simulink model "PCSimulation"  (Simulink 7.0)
settings: Solver=FixedStepDiscrete  SolverMode=SingleTasking  StartTime=0.0  StopTime=inf  FixedStep=samplePeriod  RelTol=1e-3  AbsTol=1e-6
PreLoadFcn:
  | initialize
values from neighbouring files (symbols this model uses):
  acal = acal(:)    [initialize.m]
  actParams = [	bulkModulus   * pressCanon    [initialize.m]
  atype = ones(nact, 1)    [dampmatrix.m]    (also in displA2T.m = []; displEnvelope.m = varargin{1}{6}; displJacobian.m; displT2A.m = [])
  dcal = dcal(:)    [initialize.m]
  fcal = fcal(:)    [initialize.m]
  forceCanon = 0.00444822    [initialize.m]
  inertia = inertia + inertiaP2Q([0 0 0], massA(i), cgA(:,i)-cg,  									inertiaCanon, massCanon)    [initialize.m]
  inertiaMask = zeros(3, 1)    [initialize.m]
  lengthCanon = 25.4    [initialize.m]
  mass = ones(3, 1) * (sum(massA) + massT + massS)    [initialize.m]
  massMask = zeros(3, 1)    [initialize.m]
  nAct = self.nAct    [animation.m]    (also in initialize.m = size(rh, 2))
  nAdcU = 6    [initialize.m]
  nTbl = length(dof)    [initialize.m]
  nUDPInp = 1+nTbl+2*nAct+nAcc+nAdcU    [initialize.m]
  nUDPOut = 1+5*nTbl+nAct+nAdcU    [initialize.m]
  returnPress = 50    [initialize.m]
  rtg = cg    [initialize.m]
  samplePeriod = controlPeriod/upsampleFactor    (= 0.00048828125)    [initialize.m]    (also in viewer.m = eval(getHeaderValue(header, 'DELTA_T')))
  staticForce = forceT2A(ftbl, dtbl0, dof, rh, rb, rl, canon, atype)    [initialize.m]
  upsampleFactor = 1    [initialize.m]
  x = []    [loadbin.m]    (also in quake.m = 365; viewer.m = 40; player.m = xPanel + panelWide + margin; resondemo.m = xOrigin + marginWide + panelWide + plotMarginWide)
undefined symbols (not defined in the file or in its folder): animation, DiscIntNeverNeededParam, friction, yieldDispl
libraries: LibDynamics x12, LibTransforms x12

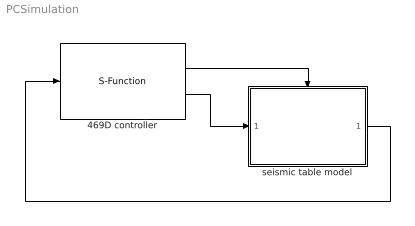
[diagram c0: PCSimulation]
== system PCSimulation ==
  469D controller : S-Function  FunctionName=UDPSimulink  Parameters=5002,nUDPInp,nUDPOut,upsampleFactor
  seismic table model : Subsystem  TreatAsAtomicUnit=on
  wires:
  469D controller/2 -> seismic table model/1(inp)
  469D controller/1 -> seismic table model/Trigger
  seismic table model/1(out) -> 469D controller/1

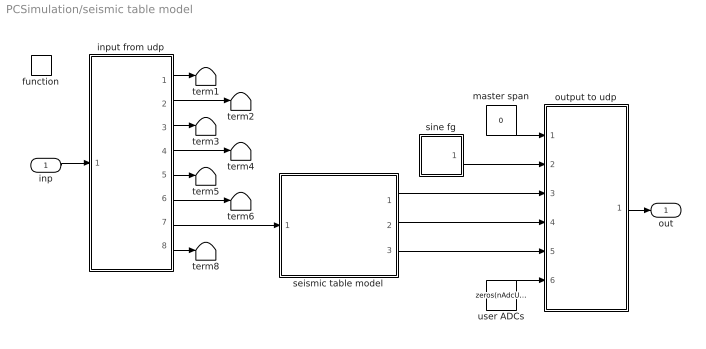
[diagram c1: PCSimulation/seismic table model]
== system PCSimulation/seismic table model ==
  inp : Inport  OutDataType=sfix(16)  OutScaling=2^0
  function : TriggerPort  TriggerType=function-call
  input from udp : Subsystem
  master span : Constant  Value=0  OutDataType=sfix(16)  OutScaling=2^0
  output to udp : Subsystem
  seismic table model : Subsystem
  sine fg : Subsystem  mask(Sine Function Generator){id=x, ampl=0.3, freq=4, phase=0, spanInterval=1, samplePeriod=-1}
      mask prompts: id "DOF"; ampl "Amplitude"; freq "Frequency (Hz)"; phase "Phase (deg)"; spanInterval "Span interval (sec)"; samplePeriod "Sample period (sec)"
  term{1..6,8} (7 alike) : Terminator
  user ADCs : Constant  Value=zeros(nAdcU, 1)  OutDataType=sfix(16)  OutScaling=2^0
  out : Outport  OutDataType=sfix(16)  OutScaling=2^0
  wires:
  input from udp/1(master span) -> term1/1
  input from udp/2(ref) -> term2/1
  input from udp/3(displ fbk) -> term3/1
  input from udp/4(veloc fbk) -> term4/1
  input from udp/5(accel fbk) -> term5/1
  input from udp/6(force fbk) -> term6/1
  input from udp/8(user adcs) -> term8/1
  input from udp/7(valve cmd) -> seismic table model/1(valve cmd)
  inp/1 -> input from udp/1(inp)
  output to udp/1(out) -> out/1
  user ADCs/1 -> output to udp/6(user adcs)
  master span/1 -> output to udp/1(master span)
  seismic table model/1(displ) -> output to udp/3(displ fbk)
  seismic table model/2(accel) -> output to udp/4(accel fbks)
  seismic table model/3(force) -> output to udp/5(force fbk)
  sine fg/1(out) -> output to udp/2(ref)

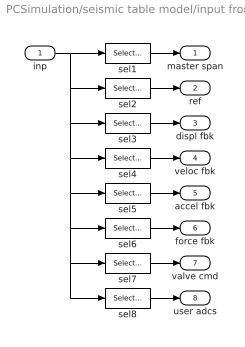
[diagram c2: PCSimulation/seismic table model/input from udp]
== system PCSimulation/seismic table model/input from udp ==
  inp : Inport  OutDataType=sfix(16)  OutScaling=2^0
  sel1 : Selector  InputPortWidth=nUDPOut  IndexOptions=Index vector (dialog)  Indices=[0]+1  OutputSizes=1
  sel2 : Selector  InputPortWidth=nUDPOut  IndexOptions=Index vector (dialog)  Indices=[1:nTbl]+1  OutputSizes=1
  sel3 : Selector  InputPortWidth=nUDPOut  IndexOptions=Index vector (dialog)  Indices=(1:nTbl)+nTbl+1  OutputSizes=1
  sel4 : Selector  InputPortWidth=nUDPOut  IndexOptions=Index vector (dialog)  Indices=(1:nTbl)+2*nTbl+1  OutputSizes=1
  sel5 : Selector  InputPortWidth=nUDPOut  IndexOptions=Index vector (dialog)  Indices=(1:nTbl)+3*nTbl+1  OutputSizes=1
  sel6 : Selector  InputPortWidth=nUDPOut  IndexOptions=Index vector (dialog)  Indices=(1:nTbl)+4*nTbl+1  OutputSizes=1
  sel7 : Selector  InputPortWidth=nUDPOut  IndexOptions=Index vector (dialog)  Indices=(1:nAct)+5*nTbl+1  OutputSizes=1
  sel8 : Selector  InputPortWidth=nUDPOut  IndexOptions=Index vector (dialog)  Indices=(1:nAdcU)+nAct+5*nTbl+1  OutputSizes=1
  master span : Outport  OutDataType=sfix(16)  OutScaling=2^0
  ref : Outport  Port=2  OutDataType=sfix(16)  OutScaling=2^0
  displ fbk : Outport  Port=3  OutDataType=sfix(16)  OutScaling=2^0
  veloc fbk : Outport  Port=4  OutDataType=sfix(16)  OutScaling=2^0
  accel fbk : Outport  Port=5  OutDataType=sfix(16)  OutScaling=2^0
  force fbk : Outport  Port=6  OutDataType=sfix(16)  OutScaling=2^0
  valve cmd : Outport  Port=7  OutDataType=sfix(16)  OutScaling=2^0
  user adcs : Outport  Port=8  OutDataType=sfix(16)  OutScaling=2^0
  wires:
  sel8/1 -> user adcs/1
  sel1/1 -> master span/1
  sel2/1 -> ref/1
  sel3/1 -> displ fbk/1
  sel4/1 -> veloc fbk/1
  sel5/1 -> accel fbk/1
  sel6/1 -> force fbk/1
  sel7/1 -> valve cmd/1
  inp/1 -> sel7/1, sel8/1, sel6/1, sel5/1, sel4/1, sel3/1, sel2/1, sel1/1

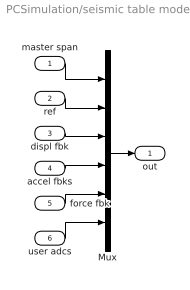
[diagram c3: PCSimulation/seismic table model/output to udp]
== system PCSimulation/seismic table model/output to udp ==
  master span : Inport  OutDataType=sfix(16)  OutScaling=2^0
  ref : Inport  Port=2  OutDataType=sfix(16)  OutScaling=2^0
  displ fbk : Inport  Port=3  OutDataType=sfix(16)  OutScaling=2^0
  accel fbks : Inport  Port=4  OutDataType=sfix(16)  OutScaling=2^0
  force fbk : Inport  Port=5  OutDataType=sfix(16)  OutScaling=2^0
  user adcs : Inport  Port=6  OutDataType=sfix(16)  OutScaling=2^0
  Mux : Mux  Inputs=6
  out : Outport  OutDataType=sfix(16)  OutScaling=2^0
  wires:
  user adcs/1 -> Mux/6
  force fbk/1 -> Mux/5
  accel fbks/1 -> Mux/4
  displ fbk/1 -> Mux/3
  ref/1 -> Mux/2
  master span/1 -> Mux/1
  Mux/1 -> out/1

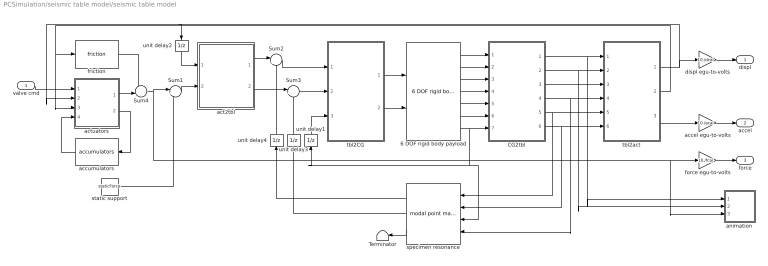
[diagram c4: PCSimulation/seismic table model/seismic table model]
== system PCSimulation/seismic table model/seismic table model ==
  valve cmd : Inport  OutDataType=sfix(16)  OutScaling=2^0
  6 DOF rigid body payload : LibDynamics/6 DOF rigid body payload  SystemSampleTime=-1  mass=mass.*massMask  inertia=diag(inertia.*inertiaMask)  gee=gee  massCanon=massCanon  inertiaCanon=inertiaCanon  linVelocCanon=linVelocCanon  linAccelCanon=linAccelCanon  rotDisplCanon=rotDisplCanon  rotVelocCanon=rotVelocCanon  rotAccelCanon=rotAccelCanon  rotForceCanon=rotForceCanon  initialPosition=zeros(6,1)  samplePeriod=samplePeriod
  CG2tbl : Subsystem  mask{ofst=-rtg}
      mask prompts: ofst "Origin offset"
  Sum1 : Sum  Inputs=|++  OutDataType=sfix(16)  OutScaling=2^0
  Sum2 : Sum  Inputs=|+-  OutDataType=sfix(16)  OutScaling=2^0
  Sum3 : Sum  Inputs=|+-  OutDataType=sfix(16)  OutScaling=2^0
  Sum4 : Sum  Inputs=-+|  OutDataType=sfix(16)  OutScaling=2^0
  Terminator : Terminator
  accel egu-to-volts : Gain  Gain=10./acal  ParameterDataType=sfix(16)  ParameterScaling=2^0  OutDataType=sfix(16)  OutScaling=2^0
  accumulators : LibDynamics/accumulators  Orientation=left  SystemSampleTime=-1  pumpFlow=pumpFlow  supplyPressure=supplyPress  precharge=precharge  bottleVolume=volume  gasConstant=gasConstant  flowCanon=flowCanon  volumeCanon=volumeCanon  samplePeriod=samplePeriod
  act2tbl : Subsystem
  actuators : Subsystem
  animation : Subsystem  mask{azim=-37.5, elev=35, params=animation, decim=ceil((1/samplePeriod)/32), samplePeriod=-1}
      mask prompts: azim "View azimuth (degrees)"; elev "View elevation (degrees)"; params "Parameters"; decim "Decimation factor"; samplePeriod "Sample period (sec)"
  displ egu-to-volts : Gain  Gain=10./dcal  ParameterDataType=sfix(16)  ParameterScaling=2^0  OutDataType=sfix(16)  OutScaling=2^0
  force egu-to-volts : Gain  Gain=10./fcal  ParameterDataType=sfix(16)  ParameterScaling=2^0  OutDataType=sfix(16)  OutScaling=2^0
  friction : LibDynamics/friction  SystemSampleTime=-1  friction=friction * forceCanon  yieldDispl=yieldDispl * lengthCanon  hysteresis=0  velocCanon=linVelocCanon  samplePeriod=samplePeriod
  specimen resonance : LibDynamics/modal point mass  Orientation=left  SystemSampleTime=-1  mass=modalMass  freq=modalFreq  damp=modalDamp  ofst=modalCG  gee=gee  massCanon=massCanon  linAccelCanon=linAccelCanon  rotDisplCanon=rotDisplCanon  rotVelocCanon=rotVelocCanon  rotForceCanon=rotForceCanon  samplePeriod=samplePeriod
  static support : Constant  Value=staticForce  OutDataType=sfix(16)  OutScaling=2^0
  tbl2CG : Subsystem  mask{ofst=rtg}
      mask prompts: ofst "Origin offset"
  tbl2act : Subsystem
  unit delay1 : UnitDelay  Orientation=up  X0=eye(3)  SampleTime=-1
  unit delay2 : UnitDelay  Orientation=down  SampleTime=-1
  unit delay3 : UnitDelay  Orientation=up  SampleTime=-1
  unit delay4 : UnitDelay  Orientation=up  SampleTime=-1
  displ : Outport  OutDataType=sfix(16)  OutScaling=2^0
  accel : Outport  Port=2  OutDataType=sfix(16)  OutScaling=2^0
  force : Outport  Port=3  OutDataType=sfix(16)  OutScaling=2^0
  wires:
  Sum4/1 -> animation/3(Fact), force egu-to-volts/1, Sum1/1
  actuators/1(force) -> Sum4/2
  friction/1 -> Sum4/1
  specimen resonance/2 -> unit delay3/1
  specimen resonance/1 -> unit delay4/1
  Sum3/1 -> tbl2CG/2(Frpw)
  act2tbl/2(Frpw) -> Sum3/1
  Sum2/1 -> tbl2CG/1(Fxyz)
  act2tbl/1(Fxyz) -> Sum2/1
  unit delay4/1 -> Sum2/2
  unit delay3/1 -> Sum3/2
  CG2tbl/6(Arpw) -> specimen resonance/2, tbl2act/6(Arpw)
  CG2tbl/5(Axyz) -> specimen resonance/1, tbl2act/5(Axyz)
  CG2tbl/4(Vrpw) -> specimen resonance/4, tbl2act/4(Vrpw)
  CG2tbl/3(Vxyz) -> tbl2act/3(Vxyz)
  CG2tbl/2(rpw) -> animation/2(rpw), tbl2act/2(rpw)
  CG2tbl/1(xyz) -> animation/1(xyz), tbl2act/1(xyz)
  tbl2act/2(veloc act) -> friction/1, actuators/3(veloc)
  unit delay2/1 -> act2tbl/1(displ act)
  unit delay1/1 -> tbl2CG/3(DCM)
  tbl2act/3(accel act) -> accel egu-to-volts/1
  6 DOF rigid body payload/7 -> specimen resonance/3, unit delay1/1, CG2tbl/7(DCM)
  6 DOF rigid body payload/6 -> CG2tbl/6(accel rpw)
  6 DOF rigid body payload/5 -> CG2tbl/5(accel xyz)
  6 DOF rigid body payload/4 -> CG2tbl/4(veloc rpw)
  6 DOF rigid body payload/3 -> CG2tbl/3(veloc xyz)
  6 DOF rigid body payload/2 -> CG2tbl/2(displ rpw)
  6 DOF rigid body payload/1 -> CG2tbl/1(displ xyz)
  tbl2CG/1(force xyz) -> 6 DOF rigid body payload/1
  valve cmd/1 -> actuators/1(cmds)
  tbl2act/1(displ act) -> displ egu-to-volts/1, actuators/2(displ), unit delay2/1
  tbl2CG/2(force rpw) -> 6 DOF rigid body payload/2
  actuators/2(flow) -> accumulators/1
  accumulators/1 -> actuators/4(press)
  force egu-to-volts/1 -> force/1
  displ egu-to-volts/1 -> displ/1
  accel egu-to-volts/1 -> accel/1
  Sum1/1 -> act2tbl/2(force act)
  static support/1 -> Sum1/2
  specimen resonance/3 -> Terminator/1

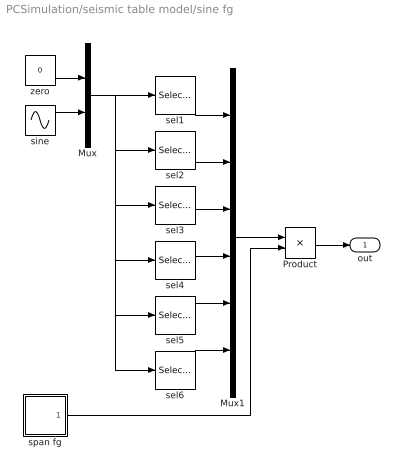
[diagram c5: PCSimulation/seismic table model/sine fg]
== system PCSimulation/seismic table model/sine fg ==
  Mux : Mux  Inputs=2
  Mux1 : Mux  Inputs=6
  Product : Product  OutDataType=sfix(16)  OutScaling=2^0
  sel1 : Selector  InputPortWidth=2  IndexOptions=Index vector (dialog)  Indices=(id==1)+1  OutputSizes=1
  sel2 : Selector  InputPortWidth=2  IndexOptions=Index vector (dialog)  Indices=(id==2)+1  OutputSizes=1
  sel3 : Selector  InputPortWidth=2  IndexOptions=Index vector (dialog)  Indices=(id==3)+1  OutputSizes=1
  sel4 : Selector  InputPortWidth=2  IndexOptions=Index vector (dialog)  Indices=(id==4)+1  OutputSizes=1
  sel5 : Selector  InputPortWidth=2  IndexOptions=Index vector (dialog)  Indices=(id==5)+1  OutputSizes=1
  sel6 : Selector  InputPortWidth=2  IndexOptions=Index vector (dialog)  Indices=(id==6)+1  OutputSizes=1
  sine : Sin  Amplitude=ampl  Frequency=2 * pi * freq  Phase=phase*180/pi  SampleTime=samplePeriod
  span fg : Subsystem  mask{spanInterval=spanInterval, samplePeriod=samplePeriod}
      mask prompts: spanInterval "Span interval (sec)"; samplePeriod "Sample period (sec)"
  zero : Constant  Value=0  OutDataType=sfix(16)  OutScaling=2^0  SampleTime=samplePeriod
  out : Outport  OutDataType=sfix(16)  OutScaling=2^0
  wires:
  span fg/1(out) -> Product/2
  Product/1 -> out/1
  Mux1/1 -> Product/1
  zero/1 -> Mux/1
  sine/1 -> Mux/2
  sel1/1 -> Mux1/1
  sel2/1 -> Mux1/2
  sel3/1 -> Mux1/3
  sel4/1 -> Mux1/4
  sel5/1 -> Mux1/5
  sel6/1 -> Mux1/6
  Mux/1 -> sel2/1, sel3/1, sel4/1, sel5/1, sel6/1, sel1/1

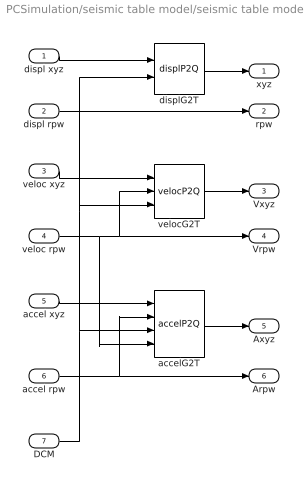
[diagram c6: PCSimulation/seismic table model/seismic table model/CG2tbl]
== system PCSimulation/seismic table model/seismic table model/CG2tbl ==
  displ xyz : Inport  OutDataType=sfix(16)  OutScaling=2^0
  displ rpw : Inport  Port=2  OutDataType=sfix(16)  OutScaling=2^0
  veloc xyz : Inport  Port=3  OutDataType=sfix(16)  OutScaling=2^0
  veloc rpw : Inport  Port=4  OutDataType=sfix(16)  OutScaling=2^0
  accel xyz : Inport  Port=5  OutDataType=sfix(16)  OutScaling=2^0
  accel rpw : Inport  Port=6  OutDataType=sfix(16)  OutScaling=2^0
  DCM : Inport  Port=7  OutDataType=sfix(16)  OutScaling=2^0
  accelG2T : LibTransforms/accelP2Q  SystemSampleTime=-1  dof=1:6  ofst=ofst
  displG2T : LibTransforms/displP2Q  SystemSampleTime=-1  dof=1:6  ofst=ofst
  velocG2T : LibTransforms/velocP2Q  SystemSampleTime=-1  dof=1:6  ofst=ofst
  xyz : Outport  OutDataType=sfix(16)  OutScaling=2^0
  rpw : Outport  Port=2  OutDataType=sfix(16)  OutScaling=2^0
  Vxyz : Outport  Port=3  OutDataType=sfix(16)  OutScaling=2^0
  Vrpw : Outport  Port=4  OutDataType=sfix(16)  OutScaling=2^0
  Axyz : Outport  Port=5  OutDataType=sfix(16)  OutScaling=2^0
  Arpw : Outport  Port=6  OutDataType=sfix(16)  OutScaling=2^0
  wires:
  accel rpw/1 -> accelG2T/2, Arpw/1
  DCM/1 -> accelG2T/3, velocG2T/3, displG2T/2
  veloc rpw/1 -> accelG2T/4, velocG2T/2, Vrpw/1
  veloc xyz/1 -> velocG2T/1
  accel xyz/1 -> accelG2T/1
  displ xyz/1 -> displG2T/1
  displG2T/1 -> xyz/1
  displ rpw/1 -> rpw/1
  velocG2T/1 -> Vxyz/1
  accelG2T/1 -> Axyz/1

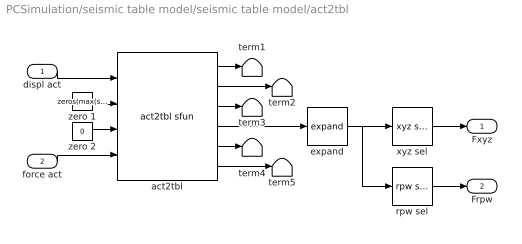
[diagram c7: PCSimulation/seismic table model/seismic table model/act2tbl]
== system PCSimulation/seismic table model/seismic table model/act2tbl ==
  displ act : Inport  OutDataType=sfix(16)  OutScaling=2^0
  force act : Inport  Port=2  OutDataType=sfix(16)  OutScaling=2^0
  act2tbl : LibTransforms/act2tbl sfun  atype=atype  nVel=0  nFrc=length(atype)  dof=dof  rh=rh  rb=rb  rl=rl  ra=[]  ea=[]  dmax=dmax  canon=canon  gee=gee  action=1  rate=0  count=1
  expand : LibTransforms/expand  SystemSampleTime=-1  size=6  elements=dof
  rpw sel : LibTransforms/rpw sel  SystemSampleTime=-1  dof=1:6
  term{1..5} (5 alike) : Terminator
  xyz sel : LibTransforms/xyz sel  SystemSampleTime=-1  dof=1:6
  zero 1 : Constant  Value=zeros(max(sum(dof>3), 1), 1)  OutDataType=sfix(16)  OutScaling=2^0
  zero 2 : Constant  Value=0  OutDataType=sfix(16)  OutScaling=2^0
  Fxyz : Outport  OutDataType=sfix(16)  OutScaling=2^0
  Frpw : Outport  Port=2  OutDataType=sfix(16)  OutScaling=2^0
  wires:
  rpw sel/1 -> Frpw/1
  force act/1 -> act2tbl/4
  xyz sel/1 -> Fxyz/1
  displ act/1 -> act2tbl/1
  act2tbl/4 -> expand/1
  zero 2/1 -> act2tbl/3
  zero 1/1 -> act2tbl/2
  act2tbl/1 -> term1/1
  act2tbl/2 -> term2/1
  act2tbl/3 -> term3/1
  act2tbl/5 -> term4/1
  act2tbl/6 -> term5/1
  expand/1 -> rpw sel/1, xyz sel/1

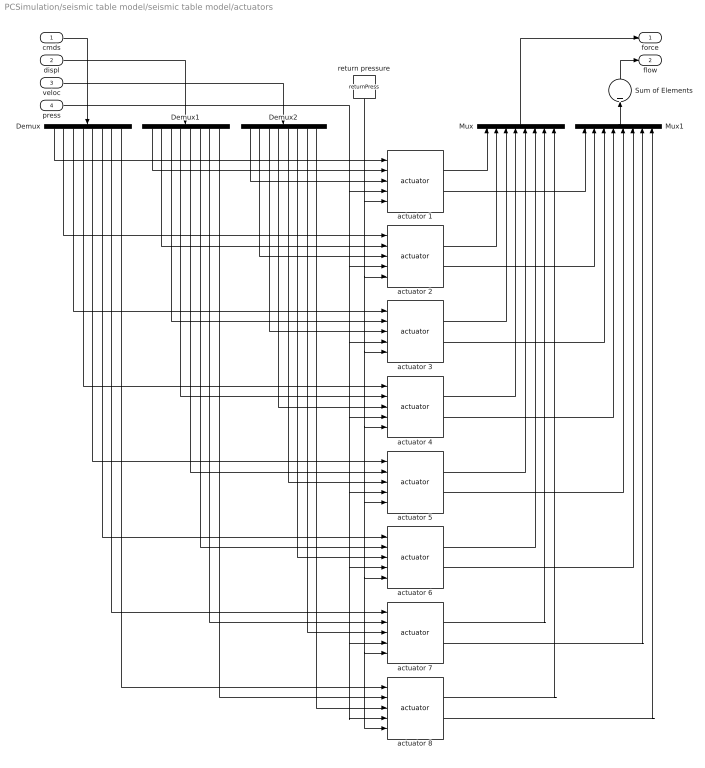
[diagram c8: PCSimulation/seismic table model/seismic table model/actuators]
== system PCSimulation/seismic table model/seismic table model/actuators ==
  cmds : Inport  OutDataType=sfix(16)  OutScaling=2^0
  displ : Inport  Port=2  OutDataType=sfix(16)  OutScaling=2^0
  veloc : Inport  Port=3  OutDataType=sfix(16)  OutScaling=2^0
  press : Inport  Port=4  OutDataType=sfix(16)  OutScaling=2^0
  Demux : Demux  Orientation=down  Outputs=nAct
  Demux1 : Demux  Orientation=down  Outputs=nAct
  Demux2 : Demux  Orientation=down  Outputs=nAct
  Mux : Mux  Orientation=up  Inputs=nAct
  Mux1 : Mux  Orientation=up  Inputs=nAct
  Sum of Elements : Sum  Orientation=up  Inputs=+  OutDataType=sfix(16)  OutScaling=2^-10
  actuator 1 : LibDynamics/actuator  SystemSampleTime=-1  params=actParams(:,1)
  actuator 2 : LibDynamics/actuator  SystemSampleTime=-1  params=actParams(:,2)
  actuator 3 : LibDynamics/actuator  SystemSampleTime=-1  params=actParams(:,3)
  actuator 4 : LibDynamics/actuator  SystemSampleTime=-1  params=actParams(:,4)
  actuator 5 : LibDynamics/actuator  SystemSampleTime=-1  params=actParams(:,5)
  actuator 6 : LibDynamics/actuator  SystemSampleTime=-1  params=actParams(:,6)
  actuator 7 : LibDynamics/actuator  SystemSampleTime=-1  params=actParams(:,7)
  actuator 8 : LibDynamics/actuator  SystemSampleTime=-1  params=actParams(:,8)
  return pressure : Constant  Orientation=down  Value=returnPress  OutDataType=sfix(16)  OutScaling=2^0
  force : Outport  OutDataType=sfix(16)  OutScaling=2^0
  flow : Outport  Port=2  OutDataType=sfix(16)  OutScaling=2^0
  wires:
  Mux/1 -> force/1
  cmds/1 -> Demux/1
  displ/1 -> Demux1/1
  Demux/1 -> actuator 1/1
  Demux/2 -> actuator 2/1
  Demux1/1 -> actuator 1/2
  Demux2/1 -> actuator 1/3
  Demux1/2 -> actuator 2/2
  Demux2/2 -> actuator 2/3
  Demux/3 -> actuator 3/1
  Demux1/3 -> actuator 3/2
  Demux2/3 -> actuator 3/3
  Demux/4 -> actuator 4/1
  Demux1/4 -> actuator 4/2
  Demux2/4 -> actuator 4/3
  Demux/5 -> actuator 5/1
  Demux1/5 -> actuator 5/2
  Demux2/5 -> actuator 5/3
  Demux/6 -> actuator 6/1
  Demux1/6 -> actuator 6/2
  Demux2/6 -> actuator 6/3
  Demux/7 -> actuator 7/1
  Demux1/7 -> actuator 7/2
  Demux2/7 -> actuator 7/3
  Demux/8 -> actuator 8/1
  Demux1/8 -> actuator 8/2
  Demux2/8 -> actuator 8/3
  actuator 1/1 -> Mux/1
  actuator 2/1 -> Mux/2
  actuator 3/1 -> Mux/3
  actuator 4/1 -> Mux/4
  actuator 5/1 -> Mux/5
  actuator 6/1 -> Mux/6
  actuator 7/1 -> Mux/7
  actuator 8/1 -> Mux/8
  veloc/1 -> Demux2/1
  press/1 -> actuator 7/4, actuator 8/4, actuator 6/4, actuator 5/4, actuator 4/4, actuator 3/4, actuator 2/4, actuator 1/4
  return pressure/1 -> actuator 7/5, actuator 8/5, actuator 6/5, actuator 5/5, actuator 4/5, actuator 3/5, actuator 2/5, actuator 1/5
  Mux1/1 -> Sum of Elements/1
  actuator 1/2 -> Mux1/1
  actuator 2/2 -> Mux1/2
  actuator 3/2 -> Mux1/3
  actuator 4/2 -> Mux1/4
  actuator 5/2 -> Mux1/5
  actuator 6/2 -> Mux1/6
  actuator 7/2 -> Mux1/7
  actuator 8/2 -> Mux1/8
  Sum of Elements/1 -> flow/1

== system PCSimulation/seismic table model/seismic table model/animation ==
  xyz : Inport
  rpw : Inport  Port=2
  Fact : Inport  Port=3
  animation : Subsystem  TreatAsAtomicUnit=on
  decimation : DiscretePulseGenerator  Period=decim  SampleTime=samplePeriod
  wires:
  decimation/1 -> animation/Trigger
  xyz/1 -> animation/1(xyz)
  Fact/1 -> animation/3(Fact)
  rpw/1 -> animation/2(rpw)

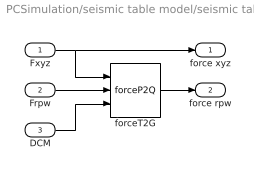
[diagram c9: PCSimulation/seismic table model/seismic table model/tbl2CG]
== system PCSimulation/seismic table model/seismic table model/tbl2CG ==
  Fxyz : Inport  OutDataType=sfix(16)  OutScaling=2^0
  Frpw : Inport  Port=2  OutDataType=sfix(16)  OutScaling=2^0
  DCM : Inport  Port=3  OutDataType=sfix(16)  OutScaling=2^0
  forceT2G : LibTransforms/forceP2Q  SystemSampleTime=-1  dof=1:6  ofst=ofst
  force xyz : Outport  OutDataType=sfix(16)  OutScaling=2^0
  force rpw : Outport  Port=2  OutDataType=sfix(16)  OutScaling=2^0
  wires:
  DCM/1 -> forceT2G/3
  forceT2G/1 -> force rpw/1
  Fxyz/1 -> force xyz/1, forceT2G/1
  Frpw/1 -> forceT2G/2

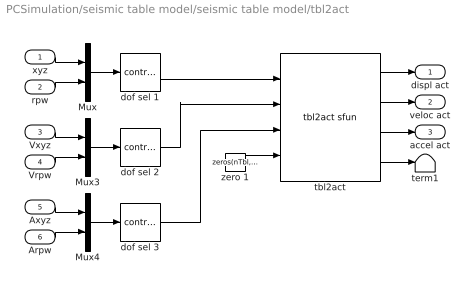
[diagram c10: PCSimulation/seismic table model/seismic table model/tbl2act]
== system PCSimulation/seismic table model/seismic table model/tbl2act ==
  xyz : Inport  OutDataType=sfix(16)  OutScaling=2^0
  rpw : Inport  Port=2  OutDataType=sfix(16)  OutScaling=2^0
  Vxyz : Inport  Port=3  OutDataType=sfix(16)  OutScaling=2^0
  Vrpw : Inport  Port=4  OutDataType=sfix(16)  OutScaling=2^0
  Axyz : Inport  Port=5  OutDataType=sfix(16)  OutScaling=2^0
  Arpw : Inport  Port=6  OutDataType=sfix(16)  OutScaling=2^0
  Mux : Mux  Inputs=2
  Mux3 : Mux  Inputs=2
  Mux4 : Mux  Inputs=2
  dof sel 1 : LibTransforms/contract  SystemSampleTime=-1  elements=dof
  dof sel 2 : LibTransforms/contract  SystemSampleTime=-1  elements=dof
  dof sel 3 : LibTransforms/contract  SystemSampleTime=-1  elements=dof
  tbl2act : LibTransforms/tbl2act sfun  atype=atype  nVel=length(atype)  nFrc=0  dof=dof  rh=rh  rb=rb  rl=rl  ra=ra  ea=ea  offset=[0 0 0 0 0 0]  fmax=fmax  canon=canon  gee=gee  action=1  rate=0
  term1 : Terminator
  zero 1 : Constant  Value=zeros(nTbl, 1)  OutDataType=sfix(16)  OutScaling=2^0
  displ act : Outport  OutDataType=sfix(16)  OutScaling=2^0
  veloc act : Outport  Port=2  OutDataType=sfix(16)  OutScaling=2^0
  accel act : Outport  Port=3  OutDataType=sfix(16)  OutScaling=2^0
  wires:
  Mux4/1 -> dof sel 3/1
  Mux3/1 -> dof sel 2/1
  Mux/1 -> dof sel 1/1
  Arpw/1 -> Mux4/2
  Axyz/1 -> Mux4/1
  Vrpw/1 -> Mux3/2
  Vxyz/1 -> Mux3/1
  rpw/1 -> Mux/2
  xyz/1 -> Mux/1
  zero 1/1 -> tbl2act/4
  tbl2act/4 -> term1/1
  tbl2act/3 -> accel act/1
  tbl2act/2 -> veloc act/1
  tbl2act/1 -> displ act/1
  dof sel 1/1 -> tbl2act/1
  dof sel 2/1 -> tbl2act/2
  dof sel 3/1 -> tbl2act/3

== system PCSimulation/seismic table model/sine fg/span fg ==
  integrator : DiscreteIntegrator  SampleTime=samplePeriod  OutDataType=sfix(16)  OutScaling=2^0  LimitOutput=on  UpperSaturationLimit=1  LowerSaturationLimit=0  ICPrevOutput=DiscIntNeverNeededParam  ICPrevScaledInput=DiscIntNeverNeededParam
  span rate : Constant  Value=1/max(spanInterval,samplePeriod)  OutDataType=sfix(16)  OutScaling=2^0  SampleTime=samplePeriod
  out : Outport  OutDataType=sfix(16)  OutScaling=2^0
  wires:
  span rate/1 -> integrator/1
  integrator/1 -> out/1

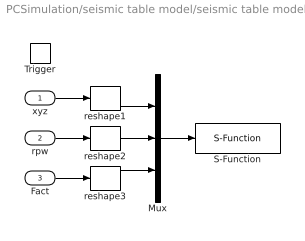
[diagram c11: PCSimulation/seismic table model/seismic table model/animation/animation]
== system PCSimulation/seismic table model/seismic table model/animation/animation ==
  xyz : Inport  OutDataType=sfix(16)  OutScaling=2^0
  rpw : Inport  Port=2  OutDataType=sfix(16)  OutScaling=2^0
  Fact : Inport  Port=3  OutDataType=sfix(16)  OutScaling=2^0
  Trigger : TriggerPort
  Mux : Mux  Inputs=3
  S-Function : S-Function  FunctionName=animation  Parameters=azim,elev,params
  reshape1 : Reshape
  reshape2 : Reshape
  reshape3 : Reshape
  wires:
  Mux/1 -> S-Function/1
  xyz/1 -> reshape1/1
  Fact/1 -> reshape3/1
  reshape3/1 -> Mux/3
  rpw/1 -> reshape2/1
  reshape2/1 -> Mux/2
  reshape1/1 -> Mux/1
